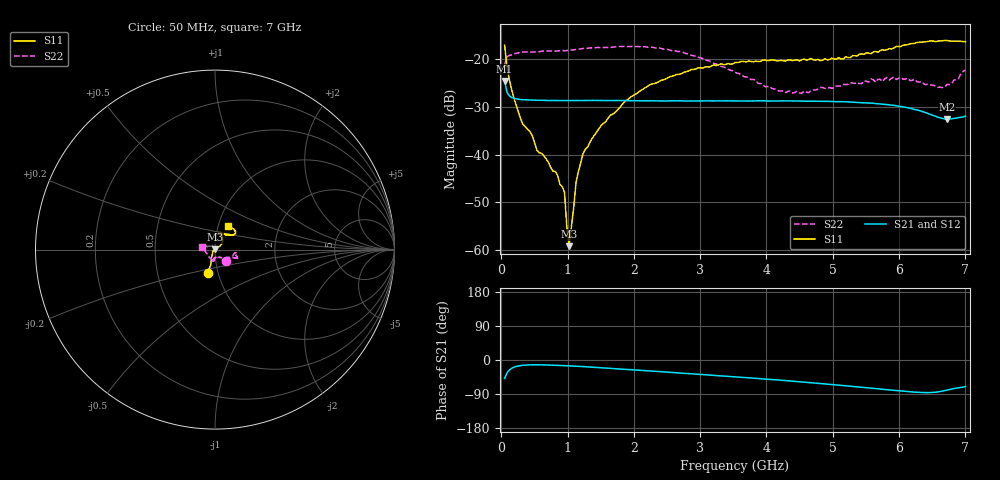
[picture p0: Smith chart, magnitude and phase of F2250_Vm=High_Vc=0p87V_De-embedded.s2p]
! Integrated Device Technology
! Corporate Headquarters
! 6024 Silver Creek Valley Road
! San Jose, CA 95138  USA
! Phone:  1-408-284-8200
! Toll Free:  1-800-223-1366
! Webpage:  http://www.idt.com/
! Timing and RF Division
! 515 Groton Road, Suite 102
! Westford, MA 01886-6024
! Device:  F2250
! Description: Voltage Variable RF Attenuator
! Frequency:  50.0 -  6000.00 MHz
! Package:  3x3 mm Thin QFN Plastic Package: 16 pin
! Ports:  2 RF, 3 DC
!  Pin  1  = GND
!  Pin  2  = NC
!  Pin  3  = RF1  = Port 1
!  Pin  4  = NC
!  Pin  5  = GND
!  Pin  6  = GND
!  Pin  7  = GND
!  Pin  8  = GND
!  Pin  9  = NC
!  Pin 10  = RF2  = Port 2
!  Pin 11  = NC
!  Pin 12  = GND
!  Pin 13  = GND
!  Pin 14  = VCNTRL
!  Pin 15  = VDD
!  Pin 16  = VMODE
! Vcntrl:  0.870 Volts
! Vmode:  +3.300 Volts
! Vdd:  +3.30  Volts
! Current:  1.311 mA
! Data:  The device was measured on a the F2250 evaluation board which has
!  individual transmission lines to the RF pins.  Data was collected
!  using a calibrated network analyzer.  The evaluation board was
!  de-embedded using a TRL calibration technique.
!  The reference plane is the edge of the package pin.
! Misc:  SN 10
!  Action Tracker AT0258
! Date Measured:  2014-11-26
! Date:  2015-10-15  MJV
! Note:
!  Integrated Device Technology supplies this data as a sample of measured
!  data at the package pin for this product.  Your particular data for this
!  product may vary.
!  Data was taken at 25 degrees C.
!  Integrated Device Technology reserves the right to change this data at anytime.
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# GHz S dB R 50
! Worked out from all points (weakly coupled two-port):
!   201 points, 50 MHz to 7 GHz, reference 50 ohm
!   highest |S21| = -24.63 dB at 50 MHz (marker M1); lowest = -32.6 dB at 6.722 GHz (marker M2)
!   lowest |S11| = -59.1 dB at 1.023 GHz (marker M3), VSWR 1.00, Z = 50 + j0.108 ohm
!   |S11| at or under -10 dB: start of sweep to end of sweep
!   |S22| runs from -27.2 to -17.4 dB; largest |S21 - S12| = 0.00011
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0.05  -17.16 -107.2  -24.63 -48.7  -24.62 -48.7  -21.26 -46.1
0.1195  -24.26 -109.8  -27.71 -26.8  -27.69 -26.8  -19.31 -13.3
0.29325  -32.62 -122.6  -28.52 -14.6  -28.52 -14.6  -18.62 -9.1
0.467  -36.03 -140.5  -28.64 -12.7  -28.62 -12.7  -18.61 -8.5
0.5365  -39.08 -147.9  -28.66 -12.7  -28.64 -12.7  -18.52 -9.6
0.84925  -44.34 172.1  -28.72 -14.1  -28.71 -14.1  -18.36 -13.9
0.9535  -47.89 176.0  -28.72 -14.9  -28.71 -14.9  -18.33 -15.1
0.98825  -55.04 171.6  -28.72 -15.2  -28.71 -15.2  -18.28 -15.5
1.023  -59.13 101.5  -28.73 -15.5  -28.71 -15.5  -18.18 -15.6
1.0925  -51.04 43.3  -28.72 -16.0  -28.73 -16.0  -18.14 -16.1
1.12725  -45.81 36.8  -28.71 -16.4  -28.73 -16.4  -18.04 -16.7
1.2315  -39.86 29.7  -28.72 -17.4  -28.71 -17.4  -17.83 -18.3
1.5095  -33.86 34.9  -28.71 -20.5  -28.73 -20.5  -17.69 -19.5
1.857  -28.99 35.9  -28.72 -24.5  -28.72 -24.5  -17.41 -21.3
2.37825  -24.74 44.6  -28.80 -30.5  -28.79 -30.5  -17.74 -22.5
2.86475  -22.24 55.8  -28.80 -36.3  -28.83 -36.3  -19.27 -24.0
3.525  -20.79 70.7  -28.80 -44.5  -28.82 -44.5  -22.80 -38.4
4.18525  -20.43 76.7  -28.82 -52.9  -28.81 -53.0  -26.75 -66.1
4.7065  -20.22 71.4  -28.86 -60.5  -28.86 -60.5  -26.49 -90.9
5.85325  -17.88 40.0  -29.64 -78.9  -29.62 -79.1  -24.42 -97.3
6.722  -16.17 48.9  -32.58 -79.1  -32.58 -79.2  -25.37 -162.1
7  -16.44 62.0  -31.95 -70.4  -31.97 -70.4  -22.37 168.4
